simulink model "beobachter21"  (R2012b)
settings: Solver=ode45  StartTime=0.0  StopTime=10.0  RelTol=1e-3
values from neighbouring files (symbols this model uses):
  A = [0 1 0 0 0 0    [beobachter_1.m]    (also in beobachter_2.m; beobachter_22.m; kalman_1.m = my_sys.a; kalman_10.m = my_sys.a)
  B = [0 1 0 0 0 0]'    [beobachter_1.m]    (also in beobachter_2.m; beobachter_22.m; kalman_1.m = my_sys.b; kalman_10.m = my_sys.b)
  C = [0 0 0 0 1 0]    [beobachter_1.m]    (also in beobachter_2.m; beobachter_22.m; kalman_1.m = my_sys.c; kalman_10.m = my_sys.c)
  D = 0    [aktiv_tilger_1.m]    (also in aktiv_tilger_12.m; aktiv_tilger_3.m = 2000; aktiv_tilger_31.m; beobachter_1.m)
  K = Kn(1:n)    [beobachter_2.m]    (also in beobachter_22.m; LQG_1.m = lqry(sys,10,1); LQR_1.m = Kn(1:6),      ki = -Kn(7),; pol_4.m)
  Ke = (place(A',C',p))'    [beobachter_1.m]    (also in beobachter_2.m; beobachter_22.m)
  ki = -Kn(n+1)    [beobachter_2.m]    (also in beobachter_22.m; kalman_12.m = -Kn(3); kalman_13.m = -Kn(4); kalman_d1.m = -Kn(4))
  x0 = [30,-20,0,0,0,0]    [beobachter_1.m]    (also in beobachter_2.m = [0,0,0,0,0.3,0]; beobachter_22.m = [0.1,0,0.1,0,0.3,0]; kalman_13.m = zeros(1,3); kalman_d1.m = zeros(1,3))

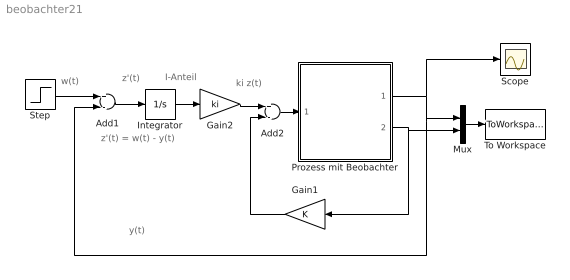
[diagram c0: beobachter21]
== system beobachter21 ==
  note: z'(t) = w(t) - y(t)
  note: y(t)
  note: w(t)
  note: ki z(t)
  note: z'(t)
  note: I-Anteil
  Add1 : Sum  Inputs=+-
  Add2 : Sum  Inputs=+-
  Gain1 : Gain  Gain=K  Multiplication=Matrix(K*u)
  Gain2 : Gain  Gain=ki
  Integrator : Integrator
  Mux : Mux  Inputs=2
  Prozess mit Beobachter : Subsystem
  Scope : Scope
  Step : Step  SampleTime=0
  To Workspace : ToWorkspace  VariableName=yx  SampleTime=-1  SaveFormat=Structure With Time
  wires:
  Add1/1 -> Integrator/1
  Step/1 -> Add1/1
  Integrator/1 -> Gain2/1
  Add2/1 -> Prozess mit Beobachter/1(u(t))
  Gain2/1 -> Add2/1
  Gain1/1 -> Add2/2
  Prozess mit Beobachter/2(GeschÃ¤tzter x(t)) -> Mux/2, Gain1/1
  Prozess mit Beobachter/1(Ausgang y(t)) -> Scope/1, Mux/1, Add1/2
  Mux/1 -> To Workspace/1

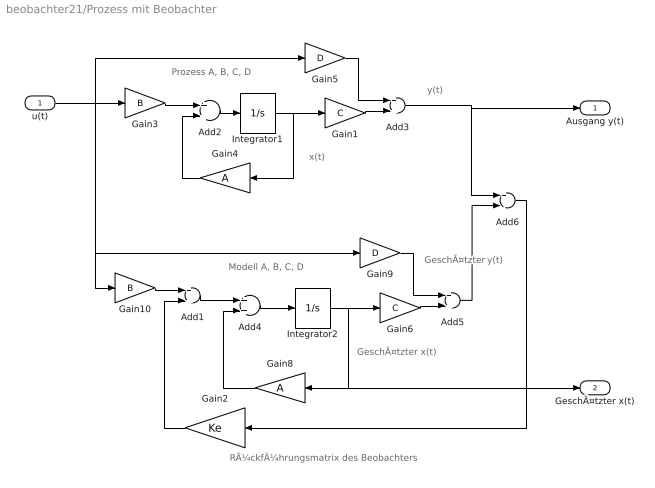
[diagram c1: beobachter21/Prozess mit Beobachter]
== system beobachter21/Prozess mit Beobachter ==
  note: Modell A, B, C, D
  note: RÃ¼ckfÃ¼hrungsmatrix des Beobachters
  note: GeschÃ¤tzter x(t)
  note: y(t)
  note: Prozess A, B, C, D
  note: x(t)
  note: y(t)
  note: GeschÃ¤tzter
  u(t) : Inport
  Add{1..5} (5 alike) : Sum
  Add6 : Sum  Inputs=+-
  Gain1 : Gain  Gain=C  Multiplication=Matrix(K*u)
  Gain10 : Gain  Gain=B  Multiplication=Matrix(K*u)
  Gain2 : Gain  Gain=Ke  Multiplication=Matrix(K*u)
  Gain3 : Gain  Gain=B  Multiplication=Matrix(K*u)
  Gain4 : Gain  Gain=A  Multiplication=Matrix(K*u)
  Gain5 : Gain  Gain=D  Multiplication=Matrix(K*u)
  Gain6 : Gain  Gain=C  Multiplication=Matrix(K*u)
  Gain8 : Gain  Gain=A  Multiplication=Matrix(K*u)
  Gain9 : Gain  Gain=D  Multiplication=Matrix(K*u)
  Integrator1 : Integrator  InitialCondition=x0
  Integrator2 : Integrator
  Ausgang y(t) : Outport
  GeschÃ¤tzter x(t) : Outport  Port=2
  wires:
  Gain2/1 -> Add1/2
  Gain10/1 -> Add1/1
  Add4/1 -> Integrator2/1
  u(t)/1 -> Gain5/1, Gain3/1, Gain9/1, Gain10/1
  Integrator2/1 -> Gain6/1, Gain8/1, GeschÃ¤tzter x(t)/1
  Gain9/1 -> Add5/1
  Gain4/1 -> Add2/2
  Gain3/1 -> Add2/1
  Add5/1 -> Add6/2
  Add6/1 -> Gain2/1
  Add2/1 -> Integrator1/1
  Gain1/1 -> Add3/2
  Gain5/1 -> Add3/1
  Add1/1 -> Add4/1
  Integrator1/1 -> Gain4/1, Gain1/1
  Add3/1 -> Add6/1, Ausgang y(t)/1
  Gain8/1 -> Add4/2
  Gain6/1 -> Add5/2
